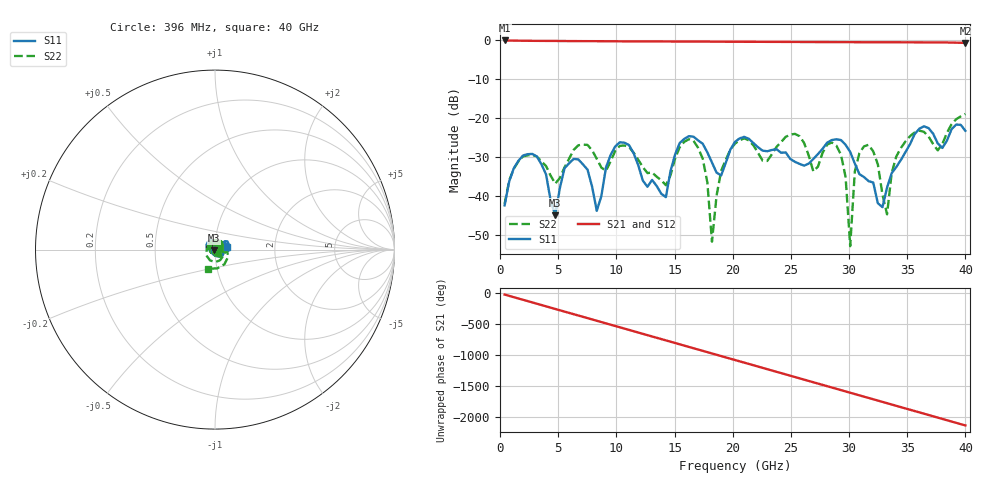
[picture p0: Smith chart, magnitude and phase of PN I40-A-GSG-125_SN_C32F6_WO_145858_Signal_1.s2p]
!  2-Port S-parameters as saved by WinCal
!VAR DATE=01-20-2010  09:17:33
!VAR OPNAME=lbui
# Hz S RI R 50.00
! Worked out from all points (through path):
!   101 points, 396 MHz to 40 GHz, reference 50 ohm
!   highest |S21| = -0.04 dB at 396 MHz (marker M1); lowest = -0.7 dB at 40 GHz (marker M2)
!   group delay of S21, straight-line fit = 148 ps
!   lowest |S11| = -44.9 dB at 4.752 GHz (marker M3), VSWR 1.01, Z = 49.6 - j0.369 ohm
!   |S11| at or under -10 dB: start of sweep to end of sweep
!   |S22| runs from -52.9 to -18.9 dB; largest |S21 - S12| = 0
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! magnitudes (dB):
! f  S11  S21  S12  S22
! 396 MHz  -42.4  0.0  0.0  -42.1
! 2.772 GHz  -29.2  -0.1  -0.1  -29.4
! 4.752 GHz  -44.9  -0.2  -0.2  -36.8
! 5.545 GHz  -32.9  -0.2  -0.2  -32.6
! 7.129 GHz  -31.9  -0.2  -0.2  -26.8
! 8.317 GHz  -43.8  -0.2  -0.2  -30.4
! 10.3 GHz  -26.2  -0.3  -0.3  -27.1
! 13.86 GHz  -39.4  -0.3  -0.3  -36.0
! 16.63 GHz  -24.8  -0.3  -0.3  -25.8
! 17.82 GHz  -28.8  -0.3  -0.3  -36.5
! 18.22 GHz  -31.4  -0.3  -0.3  -51.7
! 19.01 GHz  -34.7  -0.4  -0.4  -33.5
! 20.2 GHz  -26.1  -0.4  -0.4  -26.5
! 25.35 GHz  -31.2  -0.4  -0.4  -24.0
! 26.93 GHz  -30.5  -0.4  -0.4  -33.7
! 29.31 GHz  -25.6  -0.5  -0.5  -29.4
! 30.1 GHz  -28.7  -0.5  -0.5  -52.9
! 30.89 GHz  -34.4  -0.5  -0.5  -29.0
! 32.08 GHz  -36.5  -0.5  -0.5  -28.6
! 33.27 GHz  -37.8  -0.5  -0.5  -44.7
! 33.66 GHz  -34.1  -0.5  -0.5  -34.1
! 40 GHz  -23.3  -0.7  -0.7  -18.9
